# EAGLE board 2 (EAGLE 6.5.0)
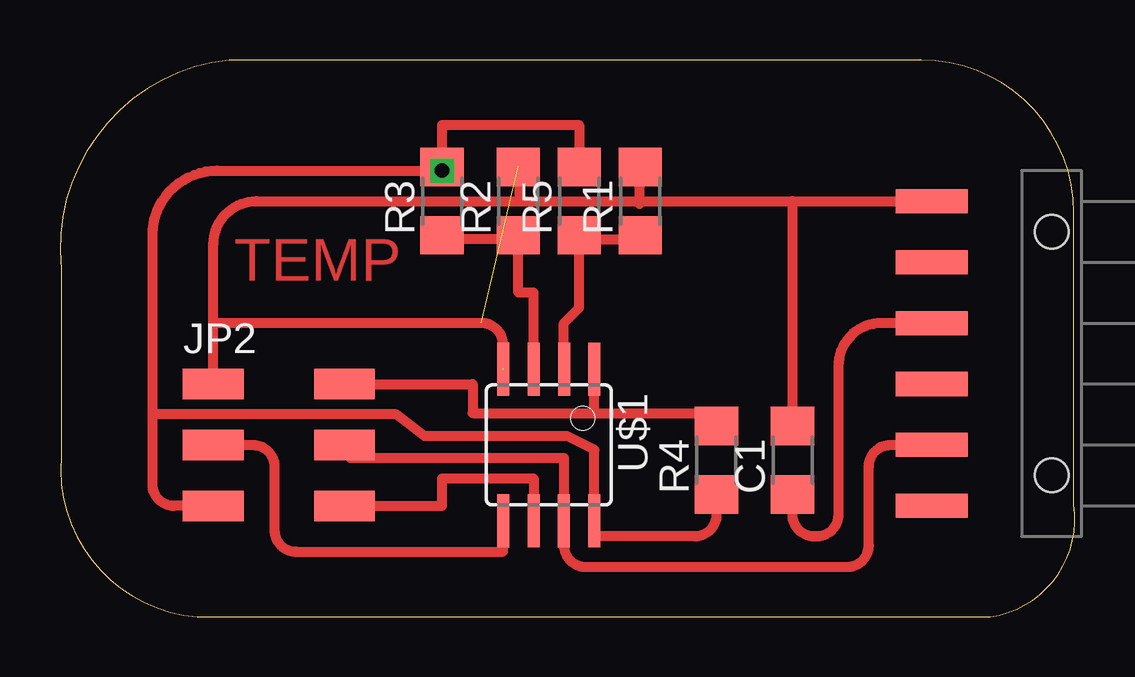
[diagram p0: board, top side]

Size 42.29 x 23.2 mm. Coordinates in mm from the lower left corner, seen from the top.
Outline: 0.04,14.5 0.04,6.67 arc90 5.71,0 38.77,0 arc90 42.24,4.68 42.24,16.83 arc90 35.88,23.2 7.05,23.2 arc90 0.04,14.5
Copper layers (1*16): Top 0.035mm / dielectric 1.5mm / Bottom 0.035mm
Design rules "default *": minimum track width 10mil, minimum drill 24mil, track to track 16mil, track to pad 16mil, pad to pad 16mil, via to via 16mil, smd to smd 16mil, copper to edge 40mil, drill to drill 16mil, minimum pad ring 10mil, minimum via ring 8mil, stop-mask expansion 4mil, vias tented up to drill 0mil, thermal gap 10mil

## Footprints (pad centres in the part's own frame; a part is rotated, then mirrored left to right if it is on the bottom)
1206 = smd 1.6 x 1.803: 1 -1.422,0; 2 1.422,0
1X06-SMD = smd 1 x 3: 1 -6.35,5; 2 -3.81,5; 3 -1.27,5; 4 1.27,5; 5 3.81,5; 6 6.35,5 | hole 1.4: -5.08,0; 5.08,0
2X03SMD = smd 2.54 x 1.27: 1 -2.54,2.54; 2 2.92,2.54; 3 -2.54,0; 4 2.92,0; 5 -2.54,-2.54; 6 2.92,-2.54
SOIC8 = smd 0.5 x 2.2: 1 -1.905,-3.154; 2 -0.645,-3.154; 3 0.625,-3.154; 4 1.895,-3.154; 5 1.905,3.154; 6 0.635,3.154; 7 -0.635,3.154; 8 -1.905,3.154

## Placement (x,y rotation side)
C1  [1206]  30.52,6.53 90 top
JP1  [1X06-SMD]  41.32,10.97 90 top
JP2  [2X03SMD]  8.93,7.16 0 top
R1  [1206]  24.17,17.32 90 top
R2  [1206]  19.09,17.32 90 top
R3  [1206]  15.92,17.32 90 top
R4  [1206]  27.35,6.53 90 top
R5  [1206]  21.63,17.32 90 top
U$1  ATTINY45SI  [SOIC8]  20.36,7.16 180 top

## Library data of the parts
C1 JP2 = 01_FAB_Hello
JP1 = 01_SparkFun
R1-R3 = ng
R4 R5 = 01_ng
U$1 = 01_fab

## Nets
N$1: JP2.3 U$1.5
N$2: JP2.5
N$3: JP2.2 U$1.1
N$5: JP2.4 U$1.7
N$6: JP2.6 U$1.6
N$8: R2.1 U$1.3
N$9: U$1.2
N$10: JP2.1 R2.2 U$1.4
N$18: R3.2

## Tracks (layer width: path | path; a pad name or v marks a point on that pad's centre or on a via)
N$1
  Top 0.406: JP2.3 8.04,7.16 arc-90 8.93,6.26 8.93,3.61 arc90 9.83,2.71 18.46,2.71 U$1.5
N$2
  Top 0.406: 21.13,7.53 15.19,7.53 14.01,8.43 3.85,8.43 | JP2.5 4.75,4.62 arc-90 3.85,5.52 3.85,8.43 | 3.85,8.43 3.85,15.9 arc-90 6.55,18.59 15.92,18.59
N$3
  Top 0.406: JP2.2 17.19,9.7 17.19,8.49 22.27,8.49 | 22.27,8.49 U$1.1 | 22.27,8.49 27.35,8.48 27.35,7.79
N$4
  Top 0.406: 21,3.35 21,2.98 arc90 21.9,2.08 32.8,2.08 arc90 33.7,2.98 33.7,6.26 arc-90 34.6,7.16 36.24,7.16
N$5
  Top 0.406: JP2.4 12.11,7.16 | 12.74,7.16 12.11,7.16 | 12.11,7.16 12.11,6.62 21,6.62 U$1.7
N$6
  Top 0.406: JP2.6 15.92,4.62 15.92,5.77 19.73,5.77 U$1.6
N$7
  Top 0.406: 36.24,12.24 34.23,12.24 arc90 32.43,10.44 32.43,4.25 arc-90 31.53,3.35 31.42,3.35 arc-90 30.52,4.25 30.52,5.26
N$8
  Top 0.406: U$1.3 19.73,10.31 19.73,13.51 19.09,13.51 19.09,15.73 | 19.09,15.73 R2.1 | 19.09,15.73 15.92,15.73
N$10  (2 unrouted)
  Top 0.406: 18.46,10.34 18.46,11.34 arc90 17.56,12.24 6.39,12.24 | JP2.1 6.39,12.24 | 6.39,12.24 6.39,15.52 arc-90 8.19,17.32 30.52,17.32 | 30.52,17.32 36.24,17.32 | 30.52,8.43 30.52,17.32
N$11
  Top 0.406: 21,10.97 21,12.24 21.63,12.88 21.63,15.73 24.17,15.73
N$12
  Top 0.406: 22.27,3.99 22.27,6.96 21.13,7.53
N$13
  Top 0.406: 19.14,18.7 19.14,17.4
N$14
  Top 0.406: 24.04,18.8 24.14,18.8 24.14,17.2
N$15
  Top 0.406: 27.35,4.62 27.35,4.25 arc-90 26.45,3.35 22.27,3.35
N$16  (via drill 0.6)
  Top 0.406: v15.92,18.59 15.92,20.5 21.63,20.5 21.63,18.59

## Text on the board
Top: TEMP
